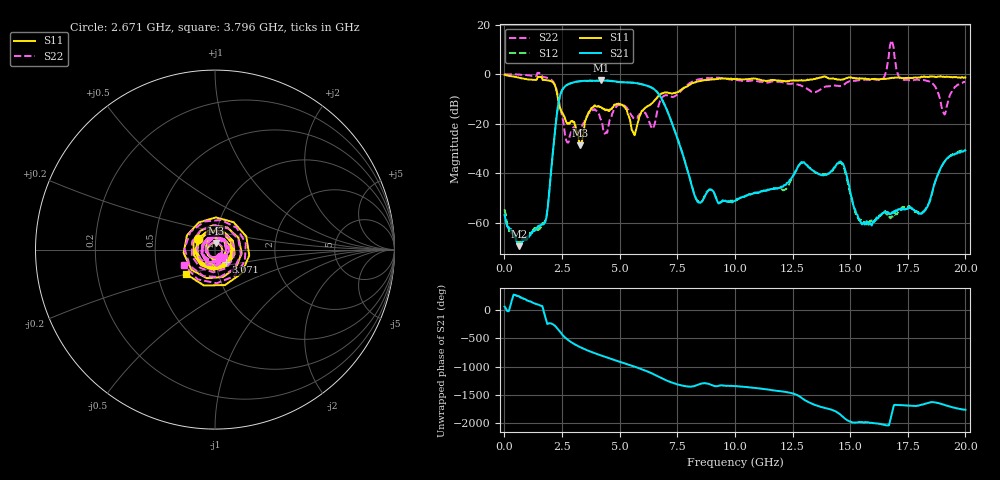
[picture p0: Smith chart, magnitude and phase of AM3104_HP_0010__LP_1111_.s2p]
!Created with skrf (http://scikit-rf.org).
# Hz S RI R 50.0
!freq ReS11 ImS11 ReS21 ImS21 ReS12 ImS12 ReS22 ImS22
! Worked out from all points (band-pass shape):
!   1601 points, 10 MHz to 20 GHz, reference 50 ohm
!   highest |S21| = -2.55 dB at 4.183 GHz (marker M1); lowest = -69.4 dB at 647.2 MHz (marker M2)
!   |S21| within 3 dB of the highest: 2.569 GHz to 6.417 GHz (3.848 GHz wide, 85.6 % of centre)
!   lowest |S11| = -28.6 dB at 3.283 GHz (marker M3), VSWR 1.08, Z = 50.3 + j3.7 ohm
!   |S11| at or under -10 dB: 2.328 GHz to 6.574 GHz (4.246 GHz wide, 95.4 % of centre)
!   |S22| runs from -27.6 to 13.6 dB; largest |S21 - S12| = 0.083
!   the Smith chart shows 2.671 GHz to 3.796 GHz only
!   S11 on the Smith chart (normalised r, x): 2.671 GHz: 0.82, +0.09; 3.071 GHz: 1.12, -0.16; 3.796 GHz: 0.70, -0.20
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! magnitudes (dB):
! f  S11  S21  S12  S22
! 10 MHz  -0.2  -56.8  -54.5  0.0
! 647.2 MHz  -1.5  -69.4  -68.2  -0.2
! 1.772 GHz  -2.4  -59.7  -59.0  -1.3
! 2.321 GHz  -9.7  -13.2  -13.2  -8.7
! 2.671 GHz  -19.0  -4.6  -4.6  -26.2
! 3.071 GHz  -20.7  -3.1  -3.1  -22.5
! 3.283 GHz  -28.6  -2.8  -2.9  -22.6
! 3.346 GHz  -27.5  -2.8  -2.8  -21.9
! 3.796 GHz  -13.5  -2.7  -2.7  -14.3
! 4.183 GHz  -13.3  -2.5  -2.6  -18.2
! 5.132 GHz  -12.4  -3.3  -3.3  -12.4
! 5.62 GHz  -24.1  -3.5  -3.5  -17.8
! 6.682 GHz  -8.8  -7.8  -7.8  -12.9
! 8.368 GHz  -3.0  -51.3  -50.9  -2.2
! 10.01 GHz  -2.0  -51.1  -51.0  -2.4
! 13.34 GHz  -2.2  -38.6  -38.7  -7.1
! 14.64 GHz  -2.2  -35.7  -36.1  -4.7
! 15.55 GHz  -1.8  -60.2  -59.5  -2.3
! 16.68 GHz  -1.7  -56.0  -57.8  7.3
! 18.18 GHz  -1.0  -55.7  -55.4  -2.4
! 19.06 GHz  -1.0  -35.7  -35.7  -15.8
! 20 GHz  -1.3  -30.8  -30.3  -3.0
